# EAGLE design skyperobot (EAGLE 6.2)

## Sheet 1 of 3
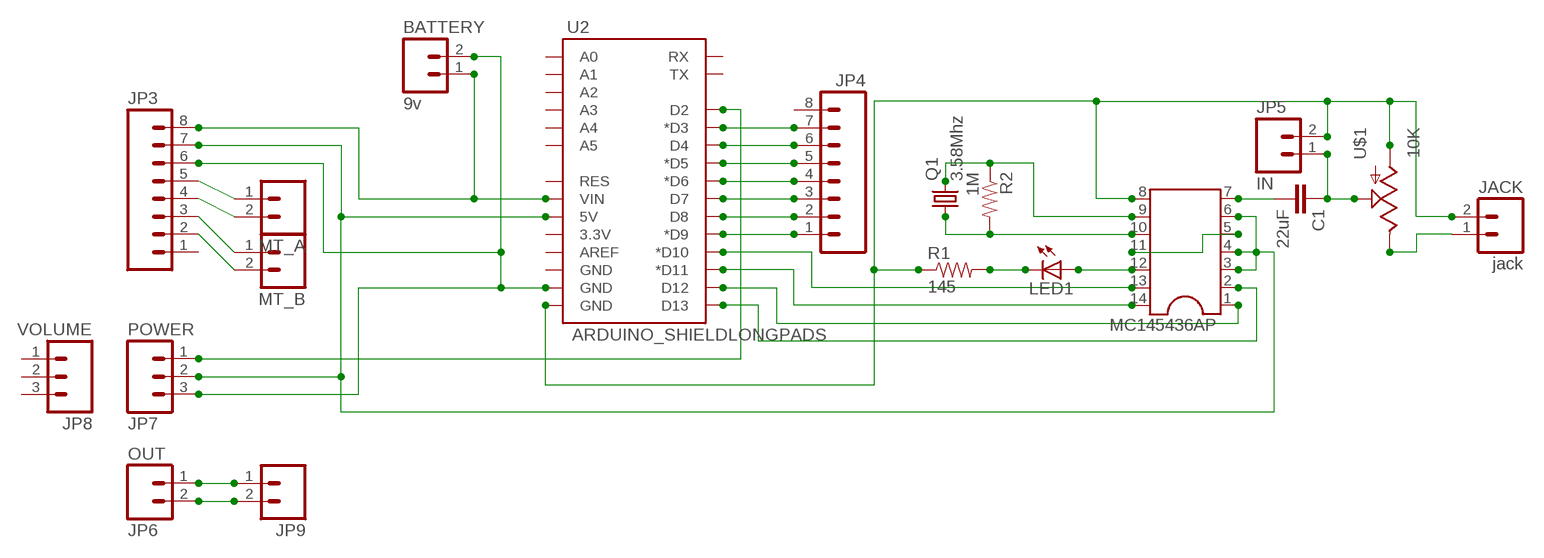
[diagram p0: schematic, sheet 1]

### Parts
BATTERY  9v  M02POLAR  [MOLEX-1X2]
C1  22uF  CAPPTH  [CAP-PTH-SMALL]
JACK  jack  M02LOCK_LONGPADS  [1X02_LOCK_LONGPADS]
JP3  M08LONGPADS  [1X08_LONGPADS]
JP4  M08LONGPADS  [1X08_LONGPADS]
JP5  IN  M02PTH  [1X02]
JP6  OUT  M02PTH  [1X02]
JP7  POWER  M03PTH  [1X03]
JP8  VOLUME  M03PTH  [1X03]
JP9  M02POLAR  [MOLEX-1X2]
LED1  LED3MM  [LED3MM]
MC145436AP  DIL14  [DIL14]
MT_A  M02POLAR  [MOLEX-1X2]
MT_B  M02POLAR  [MOLEX-1X2]
Q1  3.58Mhz  CRYSTALHC18U-H  [HC18U-H]
R1  145  RESISTORAXIAL-0.3  [AXIAL-0.3]
R2  1M  RESISTORAXIAL-0.3  [AXIAL-0.3]
U2  ARDUINO_SHIELDLONGPADS  [DUEMILANOVE_SHIELD_LONGPADS_NOHOLES]
U$1  10K  POTTRIM  [TRIM_POT_10MM]

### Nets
MT_A: JACK.2 JP5.2 MC145436AP.8 R1.P$1 U2.GND@0(GND) U$1.3(A)
N$1: MC145436AP.10 Q1.1 R2.P$2
N$2: MC145436AP.5 MC145436AP.11
N$3: JP3.7 JP7.2 MC145436AP.3 MC145436AP.4 MC145436AP.6 U2.5V
N$4 [power]: JP3.5 MT_A.1
N$5 [power]: JP3.4 MT_A.2
N$6 [power]: JP3.3 MT_B.1
N$7 [power]: JP3.2 MT_B.2
N$8: C1.2 MC145436AP.7
N$9: C1.1 JP5.1 U$1.1(S)
N$10: JP7.1 U2.D2
N$11 [power]: BATTERY.1 JP3.8 U2.VIN
N$12 [power]: BATTERY.2 JP3.6 JP7.3 U2.GND@1(GND)
N$15: LED1.K(C) R1.P$2
N$18: JP4.7 U2.D3(*D3)
N$19: JP4.6 U2.D4
N$20: JP4.5 U2.D5(*D5)
N$21: JP4.4 U2.D6(*D6)
N$22: JP4.3 U2.D7
N$23: JP4.2 U2.D8
N$24: JP4.1 U2.D9(*D9)
N$25: LED1.A MC145436AP.12
N$27: MC145436AP.1 U2.D12
N$30: JP6.1 JP9.1
N$31: JP6.2 JP9.2
N$34: MC145436AP.9 Q1.2 R2.P$1
N$39: MC145436AP.2 U2.D13
N$41: MC145436AP.14 U2.D11(*D11)
N$42: MC145436AP.13 U2.D10(*D10)
N$45: JACK.1 U$1.2(E)
Unconnected: JP3.1 JP4.8 JP8.1 JP8.2 JP8.3 U2.3.3V U2.A0 U2.A1 U2.A2 U2.A3 U2.A4 U2.A5 U2.AREF U2.GND@2(GND) U2.RES U2.RX U2.TX

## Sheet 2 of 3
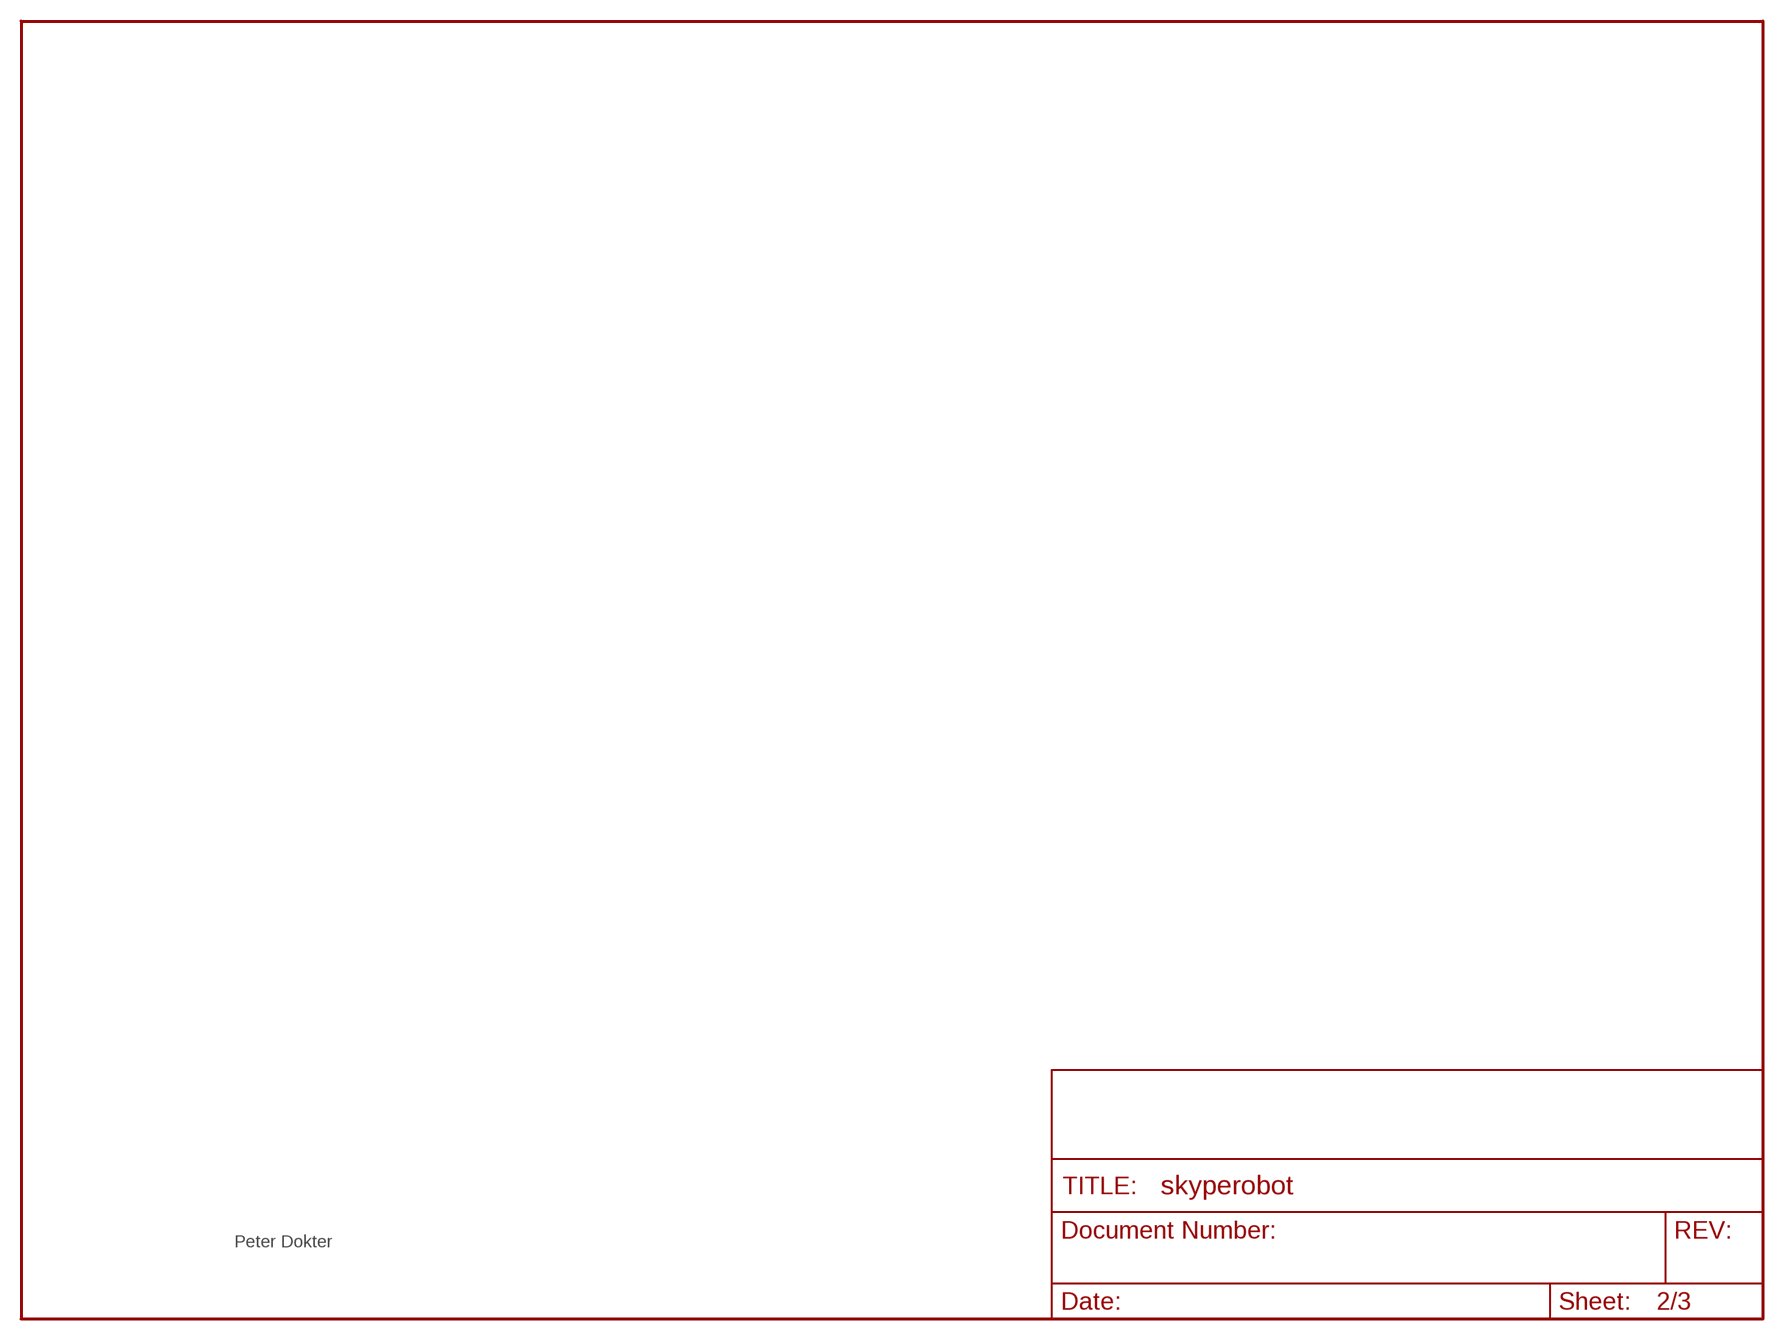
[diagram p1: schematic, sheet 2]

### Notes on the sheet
- Peter Dokter

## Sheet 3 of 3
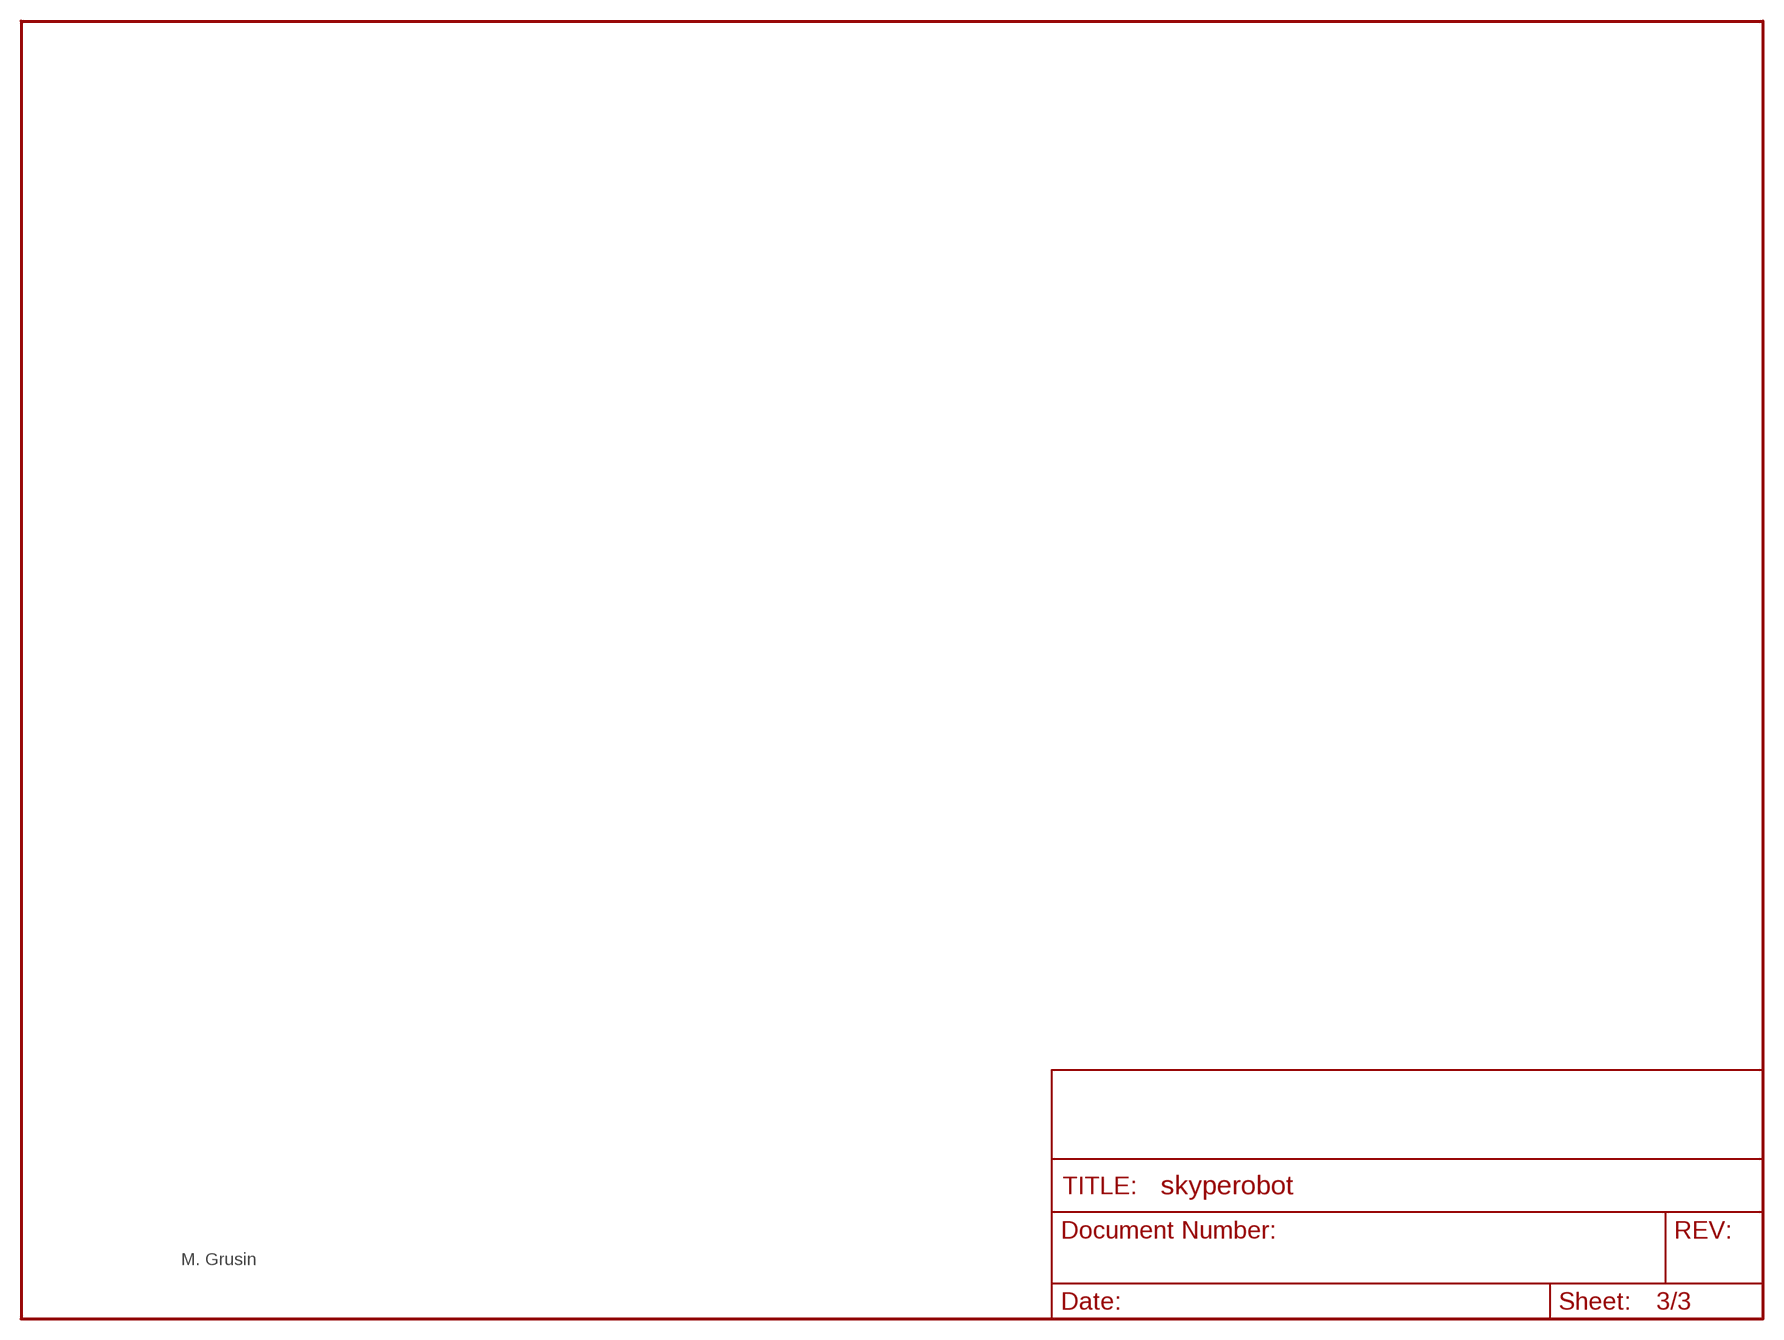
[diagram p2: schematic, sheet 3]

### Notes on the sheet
- M. Grusin

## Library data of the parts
BATTERY JACK JP5 JP6 JP9 MT_A MT_B = SparkFun:M02: Header 2
C1 = SparkFun:CAP: Capacitor
JP3 JP4 = SparkFun:M08: Header 8 Standard 8-pin 0.1" header. Use with straight break away headers (SKU : PRT-00116), right angle break away headers (PRT-00553), swiss pins (PRT-00743), machine pins (PRT-00117), and female headers (PRT-00115).
JP7 JP8 = SparkFun:M03: Header 3 Standard 3-pin 0.1" header. Use with straight break away headers (SKU : PRT-00116), right angle break away headers (PRT-00553), swiss pins (PRT-00743), machine pins (PRT-00117), and female headers (PRT-00115). Molex polarized connector foot print use with SKU : PRT-08232 with associated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
LED1 = SparkFun:LED: LEDs
MC145436AP = ic-package:DIL14: Dual In Line / Socket
Q1 = crystal:CRYSTAL: CRYSTAL; OC_FARNELL: unknown; OC_NEWARK: unknown
R1 R2 = SparkFun:RESISTOR: Resistor
U2 = SparkFun:ARDUINO_SHIELD
U$1 = SparkFun:POT

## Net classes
0 default: width 0.762 mm, clearance 0.254 mm
1 power: width 1.524 mm, clearance 0.508 mm to class 0, clearance 0.508 mm

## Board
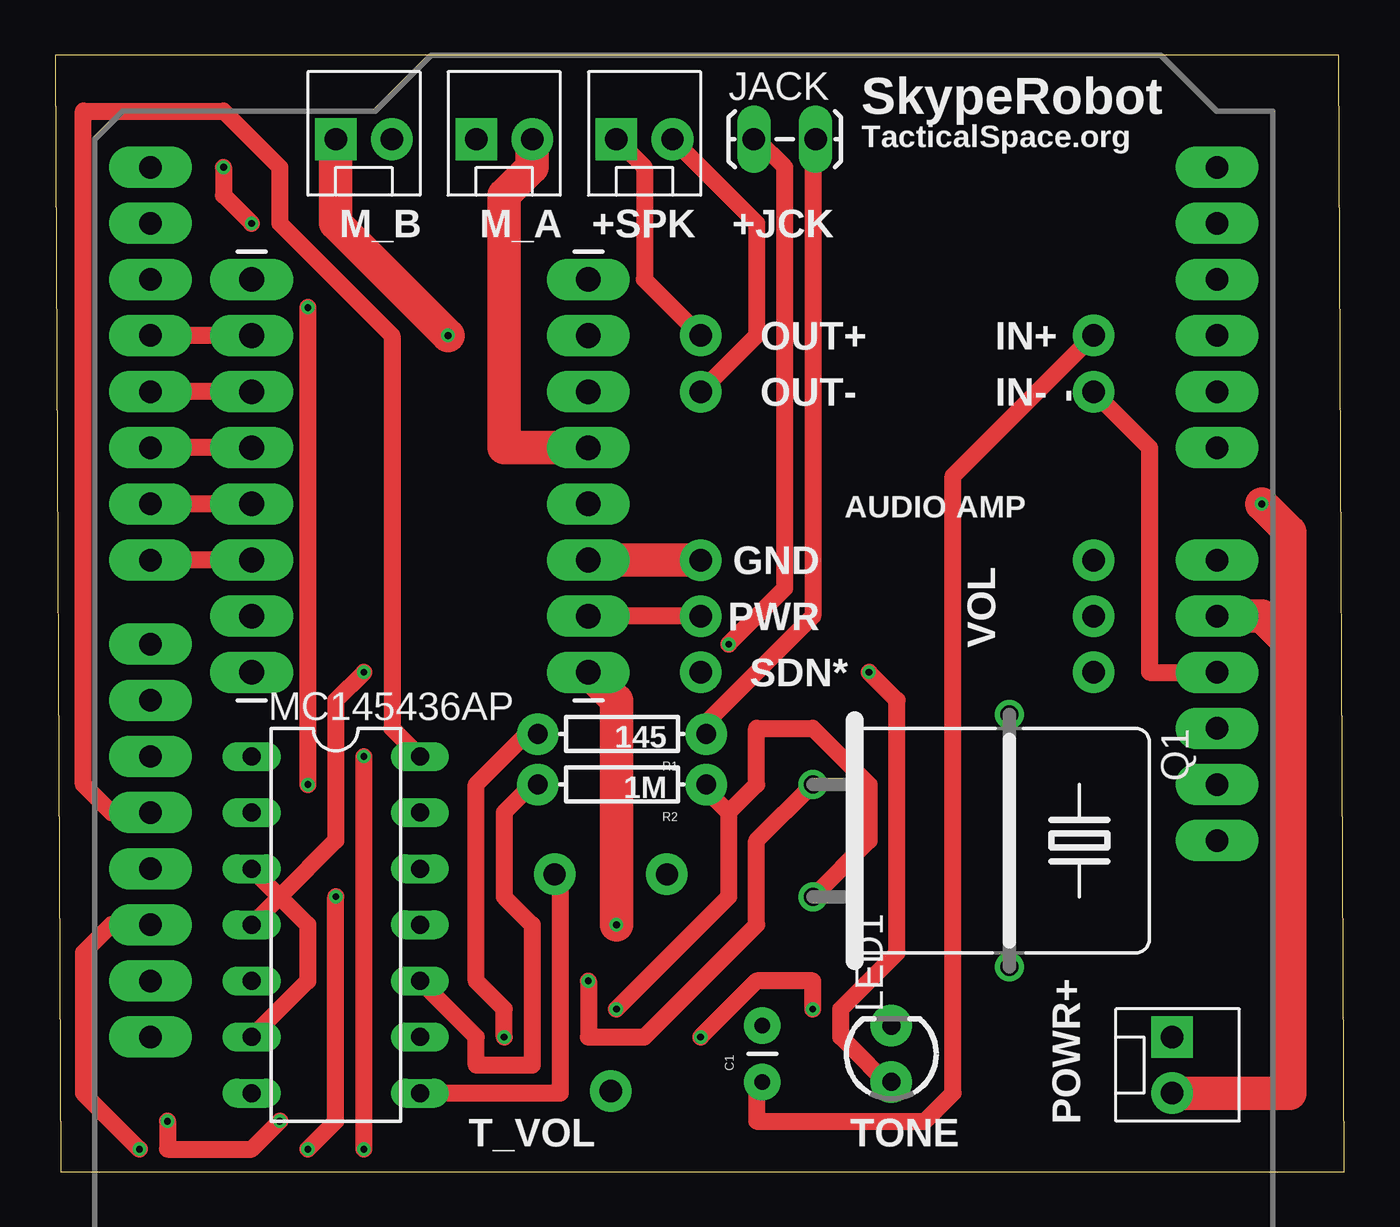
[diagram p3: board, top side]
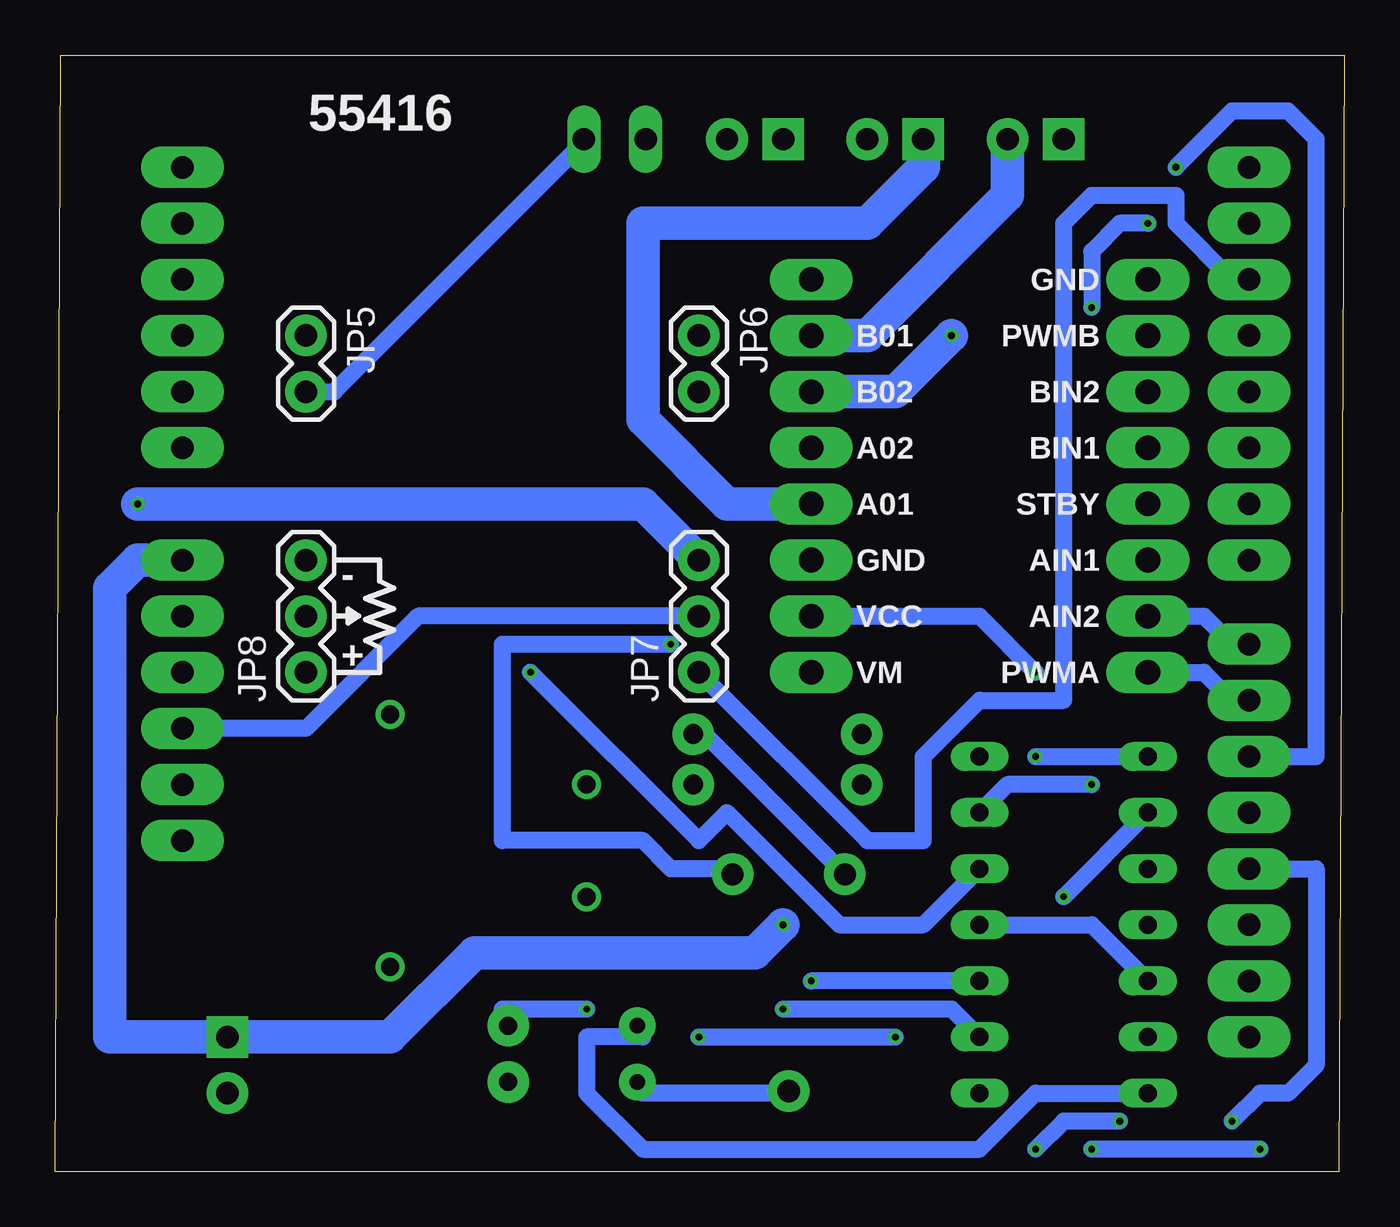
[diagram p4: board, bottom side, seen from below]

Size 58.34 x 50.54 mm. Coordinates in mm from the lower left corner, seen from the top.
Outline: 0.25,0 58.34,0 58.09,50.54 0,50.54 0.25,0
Copper layers (1*16): Top 0.035mm / dielectric 1.5mm / Bottom 0.035mm
Design rules: minimum track width 6mil, minimum drill 12mil, track to track 6mil, track to pad 6mil, pad to pad 6mil, via to via 6mil, smd to smd 0mil, copper to edge 10mil, drill to drill 10mil, minimum pad ring 10mil, minimum via ring 6mil, stop-mask expansion 2mil, vias tented up to drill 100mil, thermal gap 10mil

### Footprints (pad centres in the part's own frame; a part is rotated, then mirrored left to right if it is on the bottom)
MOLEX-1X2 = drill 1.016 pad 1.88 square: 1 0,0 | drill 1.016 pad 1.88: 2 2.54,0
CAP-PTH-SMALL = drill 0.7 pad 1.651: 1 0,0; 2 2.54,0
1X02_LOCK_LONGPADS = drill 1.016 long: 1 -0.127,0; 2 2.667,0
1X08_LONGPADS = drill 1.118 pad 1.88 long: 1 0,0; 2 2.54,0; 3 5.08,0; 4 7.62,0; 5 10.16,0; 6 12.7,0; 7 15.24,0; 8 17.78,0
1X02 = drill 1.016 pad 1.88: 1 0,0; 2 2.54,0
1X03 = drill 1.016 pad 1.88: 1 0,0; 2 2.54,0; 3 5.08,0
LED3MM = drill 0.813 pad 1.88: A -1.27,0; K 1.27,0
DIL14 = drill 0.813 long: 1 -7.62,-3.81; 2 -5.08,-3.81; 3 -2.54,-3.81; 4 0,-3.81; 5 2.54,-3.81; 6 5.08,-3.81; 7 7.62,-3.81; 8 7.62,3.81; 9 5.08,3.81; 10 2.54,3.81; 11 0,3.81; 12 -2.54,3.81; 13 -5.08,3.81; 14 -7.62,3.81
HC18U-H = drill 0.813: 1 -2.54,-5.08; 2 2.54,-5.08; M -5.715,3.81; M1 5.715,3.81
AXIAL-0.3 = drill 0.9 pad 1.88: P$1 -3.81,0; P$2 3.81,0
DUEMILANOVE_SHIELD_LONGPADS_NOHOLES = drill 1.016 pad 1.88 long: 3.3V 50.8,26.67; 5V 50.8,29.21; A0 50.8,41.91; A1 50.8,44.45; A2 50.8,46.99; A3 50.8,49.53; A4 50.8,52.07; A5 50.8,54.61; AREF 2.54,15.24; D2 2.54,49.53; D3 2.54,46.99; D4 2.54,44.45; D5 2.54,41.91; D6 2.54,39.37; D7 2.54,36.83; D8 2.54,33.02; D9 2.54,30.48; D10 2.54,27.94; D11 2.54,25.4; D12 2.54,22.86; D13 2.54,20.32; GND@0 50.8,31.75; GND@1 50.8,34.29; GND@2 2.54,17.78; RES 50.8,24.13; RX 2.54,54.61; TX 2.54,52.07; VIN 50.8,36.83
TRIM_POT_10MM = drill 1 pad 1.88: 1 9.81,0; 2 0,2.54; 3 0,-2.54

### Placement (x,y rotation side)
BATTERY  50.55,6.1 270 top
C1  32,4.06 90 top
JACK  31.75,46.74 0 top
JP3  24.13,40.39 270 top
JP4  8.89,22.61 90 top
JP5  46.99,37.85 270 bottom
JP6  29.21,37.85 270 bottom
JP7  29.21,22.61 90 bottom
JP8  46.99,22.61 90 bottom
JP9  25.4,46.74 0 top
LED1  37.85,5.33 90 top
MC145436AP  12.7,11.18 270 top
MT_A  19.05,46.74 0 top
MT_B  12.7,46.74 0 top
Q1  39.37,14.99 270 top
R1  25.65,19.81 180 top
R2  25.65,17.53 180 top
U2  1.78,-9.14 0 top
U$1  25.15,13.46 270 top

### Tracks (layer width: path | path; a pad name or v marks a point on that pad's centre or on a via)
MT_A
  Top 0.762: MC145436AP.8 22.86,3.56 22.86,13.72 U$1.3 | U2.GND@0 49.53,22.61 49.53,32.77 JP5.2 | R1.P$1 29.21,20.07 34.29,25.15 34.29,46.74 JACK.2
  Bottom 0.762: U$1.3 29.21,20.07 R1.P$1 | JP5.2 45.72,35.31 34.29,46.74 JACK.2
N$1  (via drill 0.3)
  Top 0.762: MC145436AP.10 19.05,6.1 19.05,4.83 21.59,4.83 21.59,11.18 20.32,12.45 20.32,16.26 21.59,17.53 R2.P$2 | Q1.1 31.75,14.99 31.75,11.18 26.67,6.1 24.13,6.1 v24.13,8.64
  Bottom 0.762: MC145436AP.10 v24.13,8.64
N$2
  Bottom 0.762: MC145436AP.5 11.43,11.18 MC145436AP.11
N$3  (via drill 0.3)
  Top 0.762: MC145436AP.6 11.43,8.64 11.43,11.18 10.16,12.45 | MC145436AP.3 10.16,12.45 | 10.16,12.45 MC145436AP.4 | JP7.2 JP3.7 | 10.16,12.45 12.7,14.99 12.7,21.34 v13.97,22.61
  Bottom 0.762: U2.5V 46.99,20.07 41.91,25.15 JP7.2 | v13.97,22.61 16.51,25.15 JP3.7
N$4
  Bottom 1.524: JP3.5 27.94,30.23 31.75,34.04 31.75,42.93 21.59,42.93 19.05,45.47 MT_A.1
N$5
  Top 1.524: JP3.4 20.32,32.77 20.32,44.2 21.59,45.47 MT_A.2
N$6  (via drill 0.3)
  Top 1.524: MT_B.1 12.7,42.93 v17.78,37.85
  Bottom 1.524: v17.78,37.85 20.32,35.31 JP3.3
N$7
  Bottom 1.524: JP3.2 21.59,37.85 15.24,44.2 MT_B.2
N$8
  Bottom 0.762: MC145436AP.7 13.97,3.56 16.51,1.02 31.75,1.02 34.29,3.56 34.29,6.1 31.75,6.1 C1.2
N$9
  Top 0.762: JP5.1 40.64,31.5 40.64,3.56 39.37,2.29 31.75,2.29 31.75,3.56 C1.1
  Bottom 0.762: C1.1 31.75,3.56 25.4,3.56 U$1.1
N$10
  Bottom 0.762: JP7.1 21.59,14.99 19.05,14.99 19.05,18.8 16.51,21.34 12.7,21.34 12.7,42.93 11.43,44.2 7.62,44.2 7.62,42.93 5.08,40.39 U2.D2
N$11  (via drill 0.3)
  Top 1.524: JP3.8 25.4,21.34 v25.4,11.18
  Bottom 1.524: v25.4,11.18 26.67,9.91 39.37,9.91 43.18,6.1 BATTERY.1 50.8,6.1 55.88,6.1 55.88,26.42 54.61,27.69 U2.VIN
N$12  (via drill 0.3)
  Top 1.524: JP7.3 JP3.6 | BATTERY.2 55.88,3.56 55.88,23.88 | 55.88,23.88 54.61,25.15 U2.GND@1 | v54.61,30.23 55.88,28.96 55.88,23.88
  Bottom 1.524: JP7.3 31.75,30.23 v54.61,30.23
N$15  (via drill 0.3)
  Top 0.762: v20.32,6.1 20.32,7.37 19.05,8.64 19.05,17.53 21.59,20.07 R1.P$2 | v29.21,6.1 31.75,8.64 34.29,8.64 v34.29,7.37
  Bottom 0.762: v29.21,6.1 v20.32,6.1 | v34.29,7.37 38.1,7.37 LED1.K
N$18
  Top 0.762: JP4.7 U2.D3
N$19
  Top 0.762: JP4.6 U2.D4
N$20
  Top 0.762: JP4.5 U2.D5
N$21
  Top 0.762: JP4.4 U2.D6
N$22
  Top 0.762: JP4.3 U2.D7
N$23
  Bottom 0.762: JP4.2 6.35,25.15 5.08,23.88 U2.D8
N$24
  Bottom 0.762: JP4.1 6.35,22.61 5.08,21.34 U2.D9
N$25  (via drill 0.3)
  Top 0.762: v36.83,22.61 38.1,21.34 38.1,9.91 35.56,7.37 35.56,6.1 38.1,3.56 LED1.A
  Bottom 0.762: MC145436AP.12 19.05,11.18 22.86,11.18 27.94,16.26 29.21,14.99 v36.83,22.61
N$27  (via drill 0.3)
  Top 0.762: v13.97,1.02 v13.97,18.8 | v10.16,2.29 8.89,1.02 5.08,1.02 v5.08,2.29
  Bottom 0.762: v13.97,18.8 MC145436AP.1 | v13.97,1.02 12.7,2.29 v10.16,2.29 | v5.08,2.29 3.81,3.56 2.54,3.56 1.27,4.83 1.27,13.72 U2.D12
N$30
  Top 0.762: JP6.1 26.67,40.39 26.67,45.47 JP9.1
N$31
  Top 0.762: JP6.2 31.75,37.85 31.75,42.93 JP9.2
N$34  (via drill 0.3)
  Top 0.762: v25.4,7.37 30.48,12.45 30.48,16.26 | 30.48,16.26 29.21,17.53 R2.P$1 | Q1.2 36.83,14.99 36.83,17.53 34.29,20.07 31.75,20.07 31.75,17.53 30.48,16.26
  Bottom 0.762: MC145436AP.9 17.78,7.37 v25.4,7.37
N$39  (via drill 0.3)
  Top 0.762: v12.7,12.45 12.7,2.29 v11.43,1.02 | v3.81,1.02 1.27,3.56 1.27,9.91 2.54,11.18 U2.D13
  Bottom 0.762: v12.7,12.45 MC145436AP.2 | v3.81,1.02 v11.43,1.02
N$41
  Top 0.762: MC145436AP.14 15.24,20.07 15.24,37.85 10.16,42.93 10.16,45.47 7.62,48.01 1.27,48.01 1.27,17.53 2.54,16.26 U2.D11
N$42  (via drill 0.3)
  Top 0.762: v11.43,39.12 v11.43,17.53 | v8.89,42.93 7.62,44.2 v7.62,45.47
  Bottom 0.762: MC145436AP.13 15.24,17.53 v11.43,17.53 | v11.43,39.12 11.43,41.66 10.16,42.93 v8.89,42.93 | v7.62,45.47 5.08,48.01 2.54,48.01 1.27,46.74 1.27,18.8 U2.D10
N$45  (via drill 0.3)
  Top 0.762: v30.48,23.88 33.02,26.42 33.02,45.47 31.75,46.74 JACK.1
  Bottom 0.762: v30.48,23.88 38.1,23.88 38.1,14.99 31.75,14.99 30.48,13.72 27.94,13.72 U$1.2

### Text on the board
tPlace: SkypeRobot | TacticalSpace.org | M_B | M_A | +SPK | +JCK | OUT+ | IN+ | OUT- | IN- | - | AUDIO AMP | GND | PWR | SDN* | VOL | POWR+ | T_VOL | TONE
bPlace: 55416 | GND | PWMB | B01 | BIN2 | B02 | BIN1 | A02 | STBY | A01 | AIN1 | GND | - | AIN2 | VCC | PWMA | VM | +
Measures: 0.00" | 0.05" | 0.75" | 0.80" | 0.80" | 0.55" | 0.05" | 0.00"

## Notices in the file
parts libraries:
SparkFun: Licensing: CC v3.0 Share-Alike You are welcome to use this library for commercial purposes.
